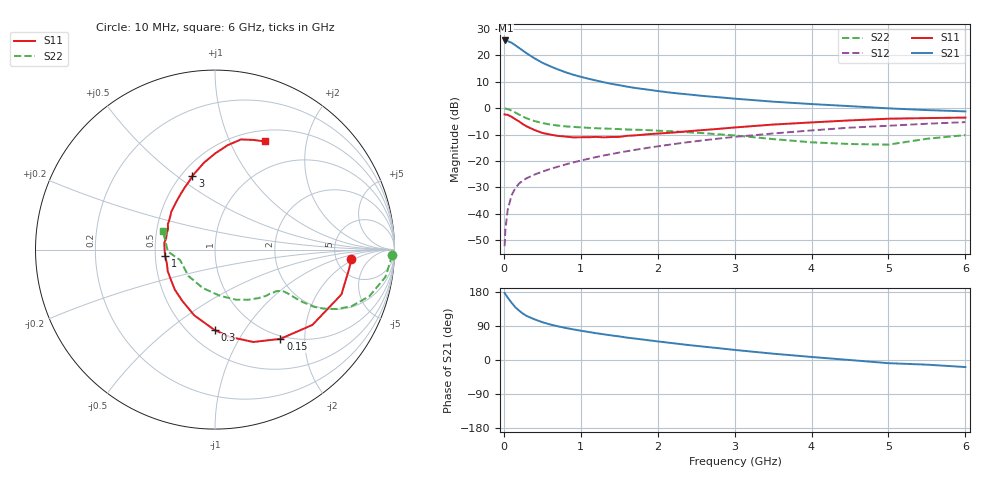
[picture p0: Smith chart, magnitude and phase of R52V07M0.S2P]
! SIEMENS Small Signal Semiconductors
! BFR183
! Si NPN RF Bipolar Junction Transistor in SOT23
! VCE = 2 V  IC = 7 mA
! Common Emitter S-Parameters:  May  1996
# GHz  S  MA  R  50
!  f  S11  S21  S12  S22
! GHz  MAG  ANG  MAG  ANG  MAG  ANG  MAG  ANG
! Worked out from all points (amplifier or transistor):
!   36 points, 10 MHz to 6 GHz, reference 50 ohm
!   highest |S21| = 25.7 dB at 20 MHz (marker M1)
!   |S21| within 3 dB of that: start of sweep to 206 MHz
!   unconditionally stable (mu >= 1): 871.8 MHz to 2.601 GHz
!   at 250 MHz: K = 0.52, MSG = 24.6 dB, |S12| = -27.4 dB
!   at 1.4 GHz: K = 1.07, MAG = 11.8 dB, |S12| = -17.4 dB
!   at 6 GHz: K = 0.89, MSG = 2.0 dB, |S12| = -5.3 dB
!   lowest NFmin = 1.25 dB at 450 MHz
!   S11 on the Smith chart (normalised r, x): 10 MHz: 6.94, -1.75; 150 MHz: 0.95, -1.53; 300 MHz: 0.66, -0.75; 1 GHz: 0.56, -0.04; 3 GHz: 0.57, +0.57; 6 GHz: 0.63, +1.36
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0.01  0.7616 -4.0  19.25 177.1  0.0024 88.8  0.9861 -1.8
0.02  0.7555 -7.9  19.3 173.6  0.0049 84.8  0.9797 -3.7
0.05  0.7475 -19.5  18.77 164.9  0.0117 81.2  0.9619 -9.1
0.1  0.6861 -37.7  17.47 151.2  0.0221 72.8  0.8985 -16.8
0.15  0.6164 -53.8  15.6 139.1  0.0305 66.3  0.8228 -22.6
0.2  0.5572 -67.5  13.86 129.9  0.0372 62.7  0.7529 -26.1
0.25  0.4942 -80.1  12.29 122.1  0.0426 60.4  0.689 -28.5
0.3  0.4487 -90.2  10.91 115.9  0.047 59.4  0.6385 -30.0
0.4  0.3842 -107.5  8.806 107.3  0.055 58.3  0.5688 -30.9
0.5  0.339 -122.5  7.29 99.8  0.0623 58.5  0.5217 -31.1
0.6  0.3159 -135.2  6.265 93.9  0.07 59.3  0.4888 -31.0
0.8  0.2895 -155.5  4.819 84.7  0.0852 60.2  0.4516 -31.3
1  0.2806 -172.7  3.941 77.3  0.1011 61.3  0.4321 -32.1
1.1  0.2808 179.8  3.621 74.0  0.1094 61.6  0.4239 -33.0
1.3  0.2795 167.1  3.103 67.8  0.1268 61.6  0.4104 -34.6
1.6  0.2986 151.5  2.566 59.1  0.1522 60.6  0.3934 -38.4
2.2  0.3439 128.5  1.947 44.3  0.2073 57.0  0.3637 -48.1
3  0.43 107.0  1.516 26.6  0.2849 49.2  0.3038 -66.9
3.5  0.4884 97.2  1.329 16.7  0.3309 43.2  0.2588 -84.0
4.5  0.5858 83.1  1.092 -0.1  0.4271 30.9  0.2087 -135.0
5.5  0.6477 70.6  0.92 -12.3  0.5066 18.6  0.2626 -177.6
6  0.6631 65.3  0.869 -18.6  0.5432 10.7  0.308 160.4
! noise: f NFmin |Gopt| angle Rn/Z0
0.45  1.25  0.18  42  0.22
0.9  1.3  0.22  110  0.2
1.8  2  0.33  180  0.14
